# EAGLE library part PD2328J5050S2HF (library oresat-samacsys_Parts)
Ultra Low Profile 0805 Power Divider Source: Datasheet
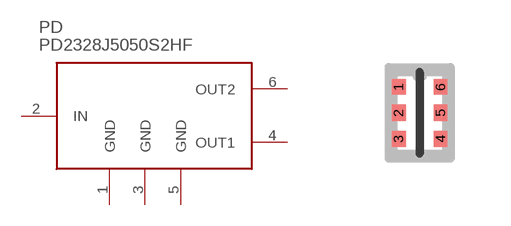
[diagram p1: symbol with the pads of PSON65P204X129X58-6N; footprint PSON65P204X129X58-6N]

Designator prefix PD

## PD2328J5050S2HF (DESCRIPTION: Ultra Low Profile 0805 Power Divider; HEIGHT: mm; MFR: ANAREN; MPN: PD2328J5050S2HF; VALUE: PD2328J5050S2HF)  [PSON65P204X129X58-6N]
1  GND  pwr
2  IN  in
3  GND  pwr
4  OUT1  out
5  GND  pwr
6  OUT2  out

## Footprint PSON65P204X129X58-6N (pad centres in mm)
EIA 481-2 (0805)
smd 0.35 x 0.4: 1 -0.525,0.65; 2 -0.525,0; 3 -0.525,-0.65; 4 0.525,-0.65; 5 0.525,0; 6 0.525,0.65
